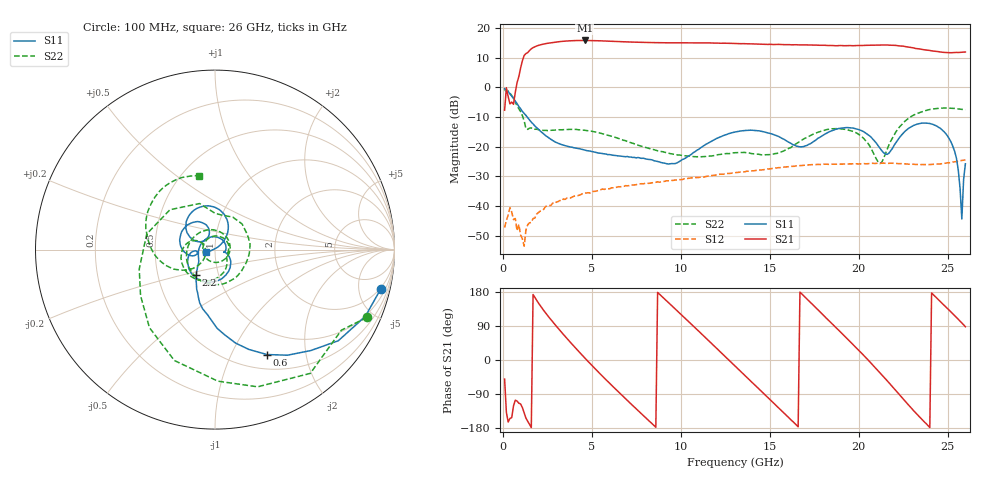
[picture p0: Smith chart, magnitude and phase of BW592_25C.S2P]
!Keysight Technologies,N5247A,US51370447,A.10.64.09
!Date: Thursday, March 05, 2020 06:25:17
!Correction: S11(Full 2 Port with power(1,2))
!S21(Full 2 Port with power(1,2))
!S12(Full 2 Port with power(1,2))
!S22(Full 2 Port with power(1,2))
!S2P File: Measurements: S11, S21, S12, S22:
# Hz S  dB  R 50
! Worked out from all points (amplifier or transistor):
!   260 points, 100 MHz to 26 GHz, reference 50 ohm
!   highest |S21| = 15.8 dB at 4.6 GHz (marker M1)
!   |S21| within 3 dB of that: 1.567 GHz to 23.56 GHz (22 GHz wide, 175 % of centre)
!   unconditionally stable (mu >= 1): start of sweep to end of sweep
!   at 4.4 GHz: K = 4.98, MAG = 16.0 dB, |S12| = -36.1 dB
!   at 13.1 GHz: K = 2.46, MAG = 15.0 dB, |S12| = -28.7 dB
!   at 26 GHz: K = 1.85, MAG = 12.9 dB, |S12| = -24.4 dB
!   S11 on the Smith chart (normalised r, x): 100 MHz: 1.83, -8.11; 600 MHz: 0.68, -1.38; 2.2 GHz: 0.78, -0.22; 26 GHz: 0.90, -0.02
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1e8  -0.45 -13.4  -7.67 -50.4  -47.26 23.3  -0.66 -24.1
6e8  -3.72 -63.7  -5.67 -121.2  -44.56 -22.9  -3.64 -110.2
1.2e9  -8.78 -96.7  10.79 -139.4  -53.50 31.1  -11.35 108.5
2.2e9  -15.19 -126.8  14.49 137.0  -41.52 4.7  -14.41 -12.3
3.3e9  -19.27 -146.4  15.52 73.1  -38.25 -26.8  -14.28 -60.2
4.5e9  -20.93 177.8  15.83 10.7  -35.70 -62.8  -14.37 -110.5
4.6e9  -21.08 174.2  15.83 5.7  -35.68 -66.6  -14.42 -114.8
6.6e9  -23.12 74.7  15.44 -88.9  -33.51 -132.1  -17.37 145.4
7.9e9  -23.87 14.3  15.19 -146.7  -32.48 -177.5  -20.00 66.2
8.8e9  -25.10 -11.8  15.08 173.8  -31.95 148.2  -21.41 4.2
1.09e10  -21.21 -25.5  15.04 81.2  -30.40 65.2  -23.36 -154.9
1.2e10  -17.25 -54.4  14.98 31.3  -29.51 19.8  -22.78 120.7
1.31e10  -14.97 -90.8  14.81 -18.2  -28.68 -27.1  -21.97 50.2
1.5e10  -15.47 -154.6  14.53 -103.4  -27.46 -104.2  -22.65 -23.8
1.63e10  -19.28 -176.3  14.38 -162.4  -26.57 -156.5  -19.71 -49.4
1.74e10  -18.54 -164.0  14.28 147.0  -26.04 158.4  -15.87 -87.3
1.91e10  -13.68 158.5  14.08 68.1  -25.84 87.4  -14.00 -157.3
2.05e10  -15.78 114.4  14.21 1.6  -25.71 26.0  -18.67 154.5
2.17e10  -22.16 141.8  14.25 -60.1  -25.58 -32.3  -19.43 -136.6
2.25e10  -15.46 151.1  13.91 -102.8  -25.72 -73.9  -11.94 -154.4
2.36e10  -12.01 113.9  12.80 -159.1  -25.99 -129.7  -8.14 166.4
2.6e10  -25.74 -167.4  11.94 87.8  -24.45 118.4  -7.55 102.1
